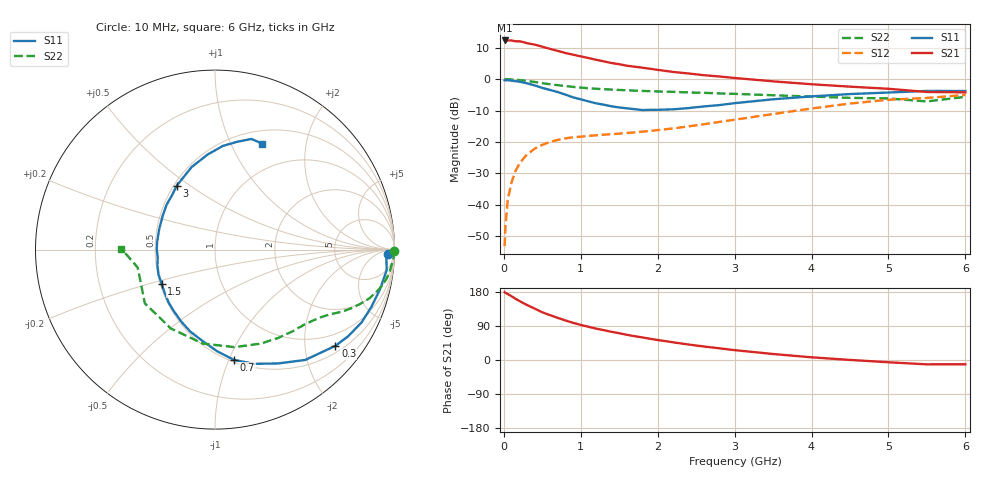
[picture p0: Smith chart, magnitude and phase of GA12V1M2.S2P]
! Infineon Technologies  Discrete & RF Semiconductors
! BF775
! Si NPN RF Bipolar Junction Transistor in SOT23
! VCE = 12 V  IC = 1.2 mA
! Common Emitter S-Parameters:  May  1996
# GHz  S  MA  R  50
!  f  S11  S21  S12  S22
! GHz  MAG  ANG  MAG  ANG  MAG  ANG  MAG  ANG
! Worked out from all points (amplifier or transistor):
!   36 points, 10 MHz to 6 GHz, reference 50 ohm
!   highest |S21| = 12.3 dB at 10 MHz (marker M1)
!   |S21| within 3 dB of that: start of sweep to 650.5 MHz
!   unconditionally stable (mu >= 1): 1.407 GHz to 3.264 GHz
!   at 250 MHz: K = 0.22, MSG = 18.6 dB, |S12| = -25.4 dB
!   at 1.4 GHz: K = 1.00, MSG = 11.3 dB, |S12| = -17.5 dB
!   at 6 GHz: K = 0.95, MSG = 0.4 dB, |S12| = -5.0 dB
!   S11 on the Smith chart (normalised r, x): 10 MHz: 39, -23; 300 MHz: 0.66, -2.71; 700 MHz: 0.52, -1.04; 1.5 GHz: 0.51, -0.22; 3 GHz: 0.52, +0.44; 6 GHz: 0.65, +1.33
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0.01  0.9628 -1.3  4.123 179.0  0.0022 83.3  0.9999 -0.4
0.02  0.9556 -2.6  4.016 177.4  0.0044 83.7  0.9963 -1.0
0.05  0.9634 -6.8  4.118 174.1  0.0119 86.0  0.9961 -2.5
0.1  0.9451 -13.7  4.12 168.3  0.0228 82.3  0.9872 -5.1
0.15  0.928 -20.1  4.002 161.7  0.0344 77.5  0.9801 -7.6
0.2  0.9121 -26.4  4.003 156.1  0.0443 74.1  0.9675 -9.9
0.3  0.859 -38.6  3.733 145.2  0.0631 67.2  0.9355 -14.1
0.4  0.7944 -50.7  3.543 135.7  0.0781 61.0  0.9014 -17.6
0.5  0.7252 -61.0  3.282 125.9  0.09 56.1  0.8613 -20.7
0.7  0.6238 -80.2  2.814 111.2  0.1079 48.8  0.8023 -25.0
0.9  0.5137 -97.8  2.448 98.1  0.1189 44.4  0.7527 -28.2
1.1  0.4423 -115.3  2.166 87.7  0.1251 42.3  0.7167 -31.0
1.3  0.3913 -131.5  1.913 78.6  0.1308 41.5  0.6905 -33.5
1.5  0.3538 -147.2  1.727 70.6  0.1357 41.9  0.6723 -36.1
1.9  0.3245 180.0  1.464 56.0  0.1497 45.4  0.6434 -41.8
2.2  0.3309 160.2  1.302 46.7  0.1642 47.7  0.6273 -46.7
3  0.4144 121.1  1.043 26.0  0.2262 51.5  0.5831 -63.9
3.5  0.478 105.8  0.922 15.8  0.2785 49.8  0.5542 -78.7
4.5  0.5791 85.7  0.759 0.2  0.4086 39.5  0.5036 -119.1
5  0.6121 78.6  0.702 -6.0  0.4699 31.5  0.4926 -142.5
5.5  0.6489 71.8  0.625 -11.5  0.502 21.7  0.4419 -166.9
6  0.6466 65.9  0.616 -11.3  0.5603 16.6  0.5219 179.4
